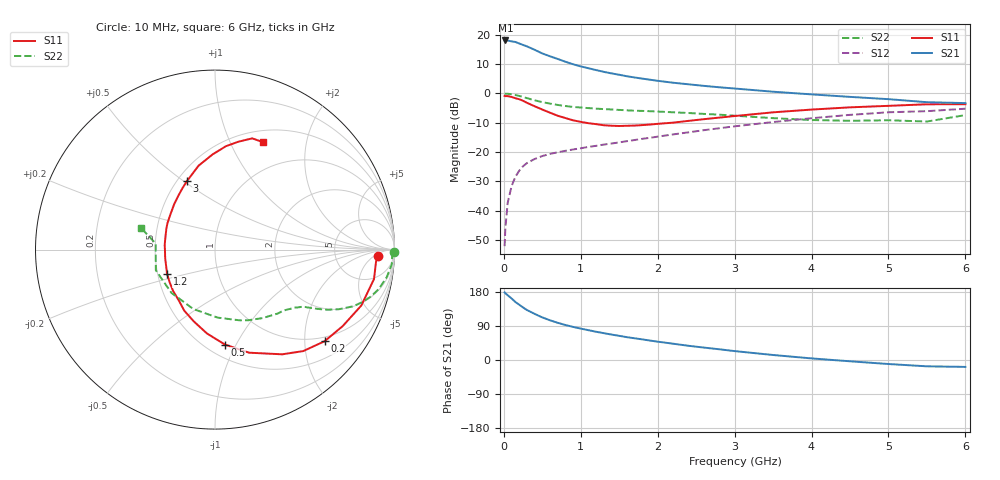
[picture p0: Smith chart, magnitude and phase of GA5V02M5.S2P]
! Infineon Technologies  Discrete & RF Semiconductors
! BF775
! Si NPN RF Bipolar Junction Transistor in SOT23
! VCE = 5 V  IC = 2.5 mA
! Common Emitter S-Parameters:  May  1996
# GHz  S  MA  R  50
!  f  S11  S21  S12  S22
! GHz  MAG  ANG  MAG  ANG  MAG  ANG  MAG  ANG
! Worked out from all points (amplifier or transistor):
!   36 points, 10 MHz to 6 GHz, reference 50 ohm
!   highest |S21| = 18.1 dB at 20 MHz (marker M1)
!   |S21| within 3 dB of that: start of sweep to 384.7 MHz
!   unconditionally stable (mu >= 1): 1.113 GHz to 3.4 GHz
!   at 250 MHz: K = 0.32, MSG = 20.7 dB, |S12| = -24.8 dB
!   at 1.4 GHz: K = 1.10, MAG = 10.0 dB, |S12| = -17.1 dB
!   at 6 GHz: K = 0.96, MSG = 1.0 dB, |S12| = -5.2 dB
!   S11 on the Smith chart (normalised r, x): 10 MHz: 18, -7; 200 MHz: 0.89, -2.48; 500 MHz: 0.61, -0.90; 1.2 GHz: 0.56, -0.17; 3 GHz: 0.56, +0.51; 6 GHz: 0.64, +1.34
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0.01  0.9072 -2.2  7.896 178.4  0.0025 90.3  0.9973 -0.9
0.02  0.8999 -4.2  7.994 176.1  0.0051 87.4  0.9881 -1.8
0.05  0.9009 -10.5  7.972 171.0  0.0137 83.6  0.9885 -4.7
0.15  0.8295 -30.9  7.534 153.1  0.038 72.1  0.9397 -13.4
0.2  0.7959 -39.9  7.099 145.9  0.0483 68.1  0.9067 -16.8
0.25  0.7492 -49.0  6.695 138.6  0.0576 63.9  0.87 -19.7
0.3  0.6933 -57.3  6.343 131.9  0.0651 60.7  0.8322 -22.3
0.4  0.605 -71.7  5.544 121.7  0.0764 55.6  0.7642 -25.8
0.5  0.532 -84.0  4.803 112.4  0.0858 52.3  0.7115 -28.1
0.6  0.4699 -95.4  4.295 104.8  0.0933 50.3  0.6712 -29.6
0.7  0.417 -106.5  3.87 98.2  0.0994 49.4  0.6368 -30.9
0.8  0.3811 -116.7  3.472 92.4  0.1053 48.8  0.6105 -31.9
0.9  0.3484 -125.2  3.144 87.3  0.111 48.7  0.5892 -32.7
1.1  0.3111 -144.4  2.688 78.7  0.1228 48.9  0.5629 -34.9
1.2  0.2998 -153.0  2.5 74.5  0.1281 49.2  0.5509 -35.9
1.6  0.2814 174.7  1.962 60.2  0.1538 50.8  0.5158 -40.9
2.2  0.3179 141.0  1.523 43.0  0.2005 51.1  0.4774 -51.0
3  0.412 112.4  1.213 23.5  0.2754 47.3  0.418 -70.6
3.5  0.4768 101.0  1.07 13.2  0.3255 42.8  0.3794 -87.7
4.5  0.5797 83.9  0.874 -3.4  0.4316 30.8  0.3422 -135.2
5.5  0.6536 71.5  0.709 -16.7  0.4989 14.9  0.3322 174.1
6  0.6557 65.9  0.685 -18.2  0.5495 10.5  0.428 163.8
